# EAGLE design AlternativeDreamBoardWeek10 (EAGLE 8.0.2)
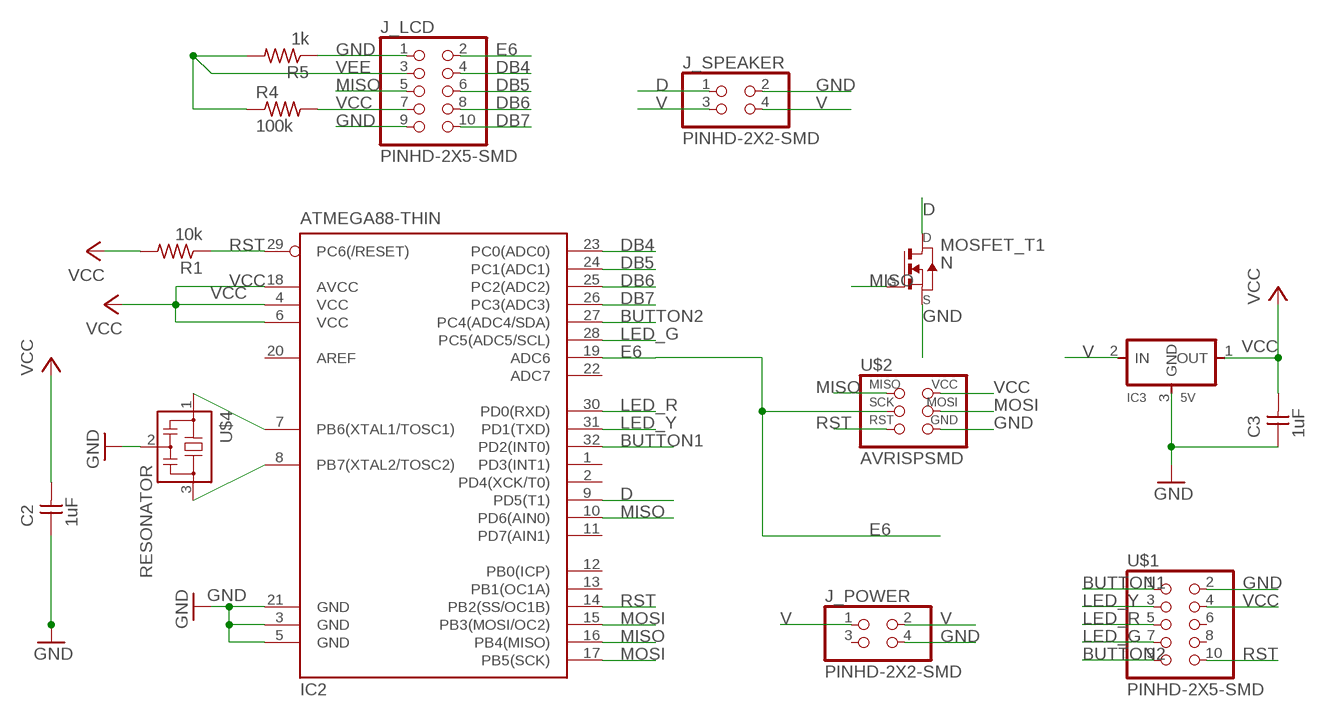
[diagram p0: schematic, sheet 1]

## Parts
C2  1uF  CAP-UNPOLARIZEDFAB  [C1206FAB]
C3  1uF  CAP-UNPOLARIZEDFAB  [C1206FAB]
IC2  ATMEGA88-THIN  [TQFP32-08THIN]
IC3  5V  REGULATORSOT23  [SOT23]
J_LCD  PINHD-2X5-SMD  [2X05SMD]
J_POWER  PINHD-2X2-SMD  [2X02SMD]
J_SPEAKER  PINHD-2X2-SMD  [2X02SMD]
MOSFET_T1  N  NMOSFETSOT23  [SOT-23]
R1  10k  RES-US1206FAB  [R1206FAB]
R4  100k  RES-US1206FAB  [R1206FAB]
R5  1k  RES-US1206FAB  [R1206FAB]
U$1  PINHD-2X5-SMD  [2X05SMD]
U$2  AVRISPSMD  [2X03SMD]
U$4  RESONATOR  [EFOBM]

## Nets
BUTTON1: IC2.32(PD2(INT0)) U$1.1
BUTTON2: IC2.27(PC4(ADC4/SDA)) U$1.9
D: IC2.9(PD5(T1)) J_SPEAKER.1 MOSFET_T1.1(D)
DB4: IC2.23(PC0(ADC0)) J_LCD.4
DB5: IC2.24(PC1(ADC1)) J_LCD.6
DB6: IC2.25(PC2(ADC2)) J_LCD.8
DB7: IC2.26(PC3(ADC3)) J_LCD.10
E6: IC2.19(ADC6) J_LCD.2 U$2.3(SCK)
GND: C2.1 C3.1 IC2.3(GND) IC2.5(GND) IC2.21(GND) IC3.3(GND) J_LCD.1 J_LCD.9 J_POWER.4 J_SPEAKER.2 MOSFET_T1.2(S) R5.1 U$1.2 U$2.6(GND) U$4.2
LED_G: IC2.28(PC5(ADC5/SCL)) U$1.7
LED_R: IC2.30(PD0(RXD)) U$1.5
LED_Y: IC2.31(PD1(TXD)) U$1.3
MISO: IC2.10(PD6(AIN0)) IC2.16(PB4(MISO)) J_LCD.5 MOSFET_T1.3(G) U$2.1(MISO)
MOSI: IC2.15(PB3(MOSI/OC2)) IC2.17(PB5(SCK)) U$2.4(MOSI)
N$1: IC2.8(PB7(XTAL2/TOSC2)) U$4.3
N$2: IC2.7(PB6(XTAL1/TOSC1)) U$4.1
RST: IC2.14(PB2(SS/OC1B)) IC2.29(PC6(/RESET)) R1.1 U$1.10 U$2.5(RST)
V: IC3.2(IN) J_POWER.1 J_POWER.2 J_SPEAKER.3 J_SPEAKER.4
VCC: C2.2 C3.2 IC2.4(VCC) IC2.6(VCC) IC2.18(AVCC) IC3.1(OUT) J_LCD.7 R1.2 R4.2 U$1.4 U$2.2(VCC)
VEE: J_LCD.3 R4.1 R5.2
Unconnected: IC2.1(PD3(INT1)) IC2.2(PD4(XCK/T0)) IC2.11(PD7(AIN1)) IC2.12(PB0(ICP)) IC2.13(PB1(OC1A)) IC2.20(AREF) IC2.22(ADC7) J_POWER.3 U$1.6 U$1.8

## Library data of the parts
C2 C3 = fab:CAP-UNPOLARIZED
IC2 = fab:ATMEGA88-THIN
IC3 = fab:REGULATOR
J_LCD U$1 = fab:PINHD-2X5-SMD
J_POWER J_SPEAKER = fab:PINHD-2X2-SMD
MOSFET_T1 = fab:NMOSFET: MOS FET
R1 R4 R5 = fab:RES-US: Resistor (US Symbol)
U$2 = fab:AVRISP
U$4 = fab:RESONATOR

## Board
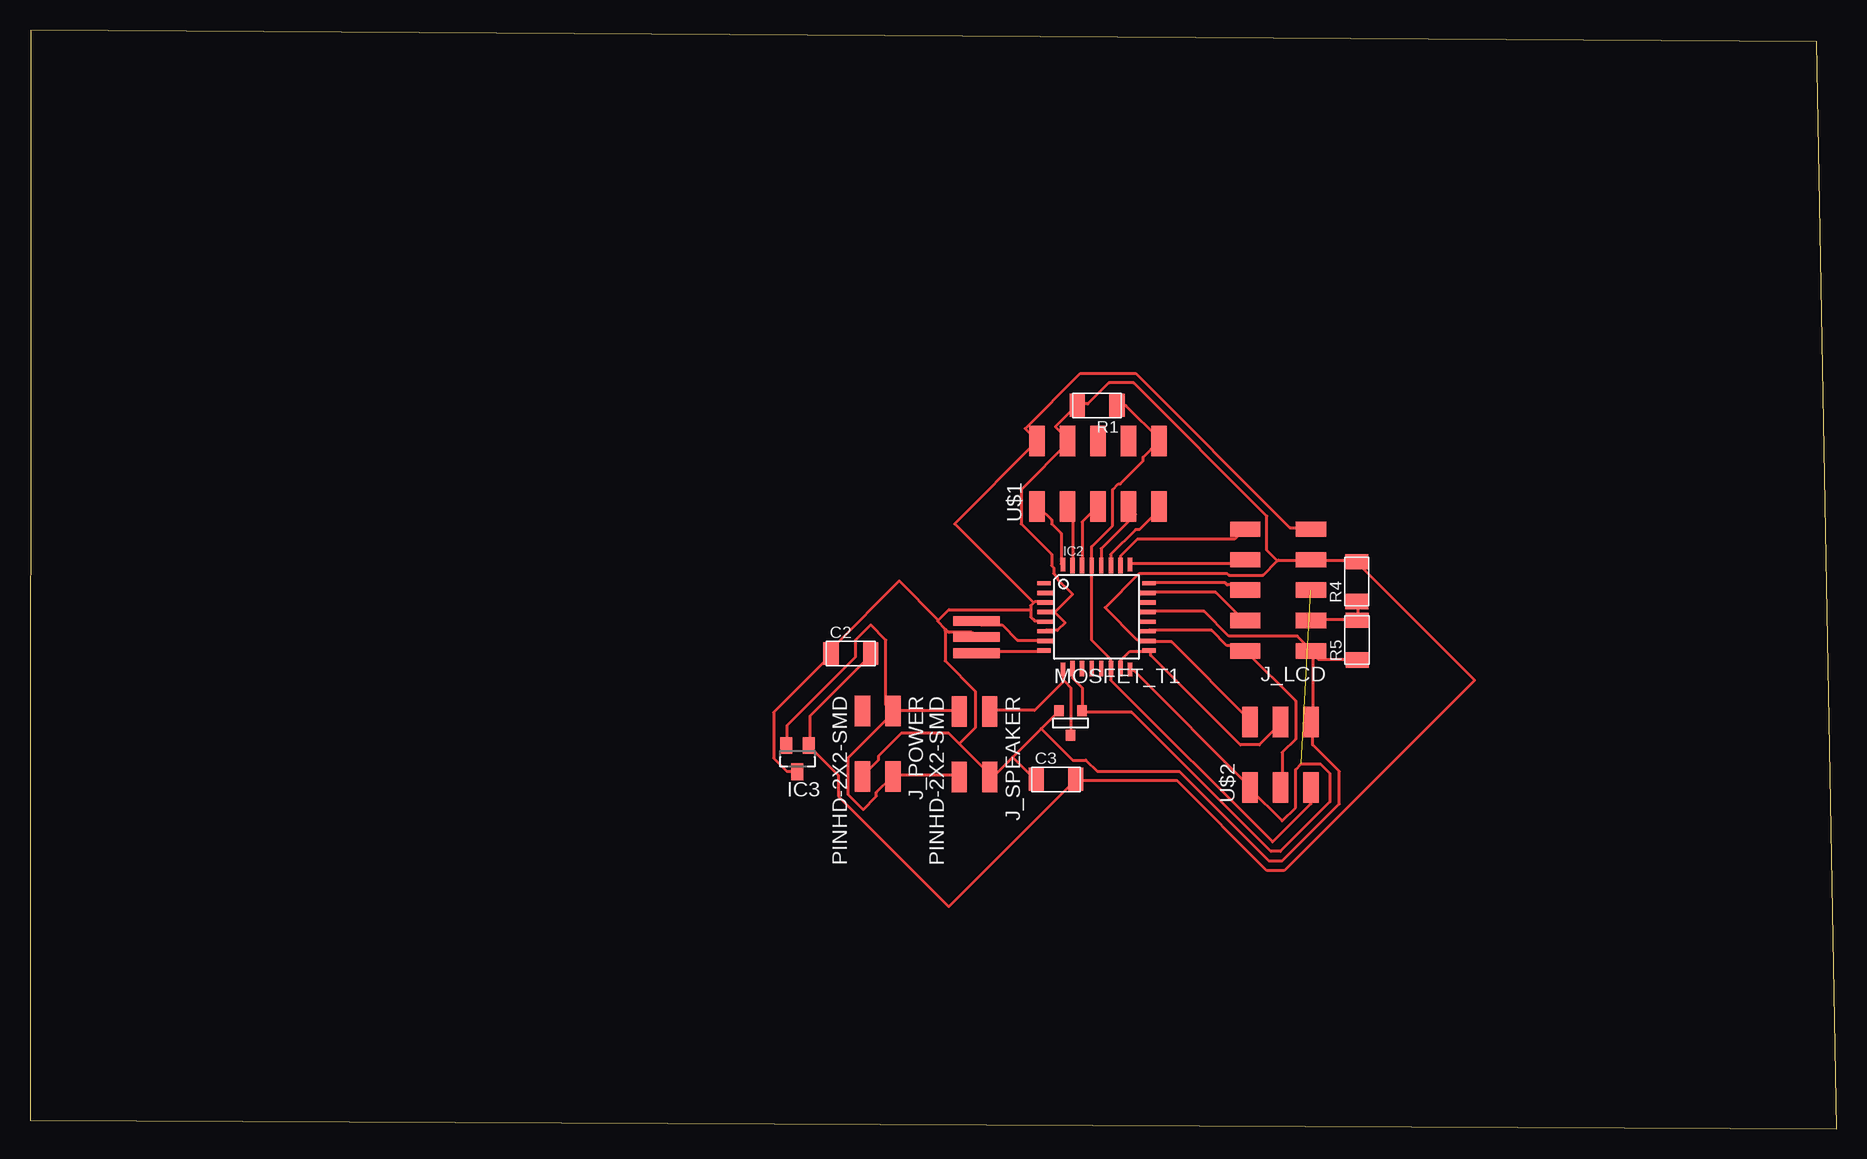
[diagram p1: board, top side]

Size 150.55 x 91.58 mm. Coordinates in mm from the lower left corner, seen from the top.
Outline: 0,0.71 150.55,0 148.89,90.62 0.08,91.58 0,0.71
Copper layers (1*16): Top 0.035mm / dielectric 1.5mm / Bottom 0.035mm
Design rules "default *": minimum track width 10mil, minimum drill 24mil, track to track 16mil, track to pad 16mil, pad to pad 16mil, via to via 16mil, smd to smd 8mil, copper to edge 40mil, drill to drill 8mil, minimum pad ring 10mil, minimum via ring 8mil, stop-mask expansion 4mil, vias tented up to drill 0mil, thermal gap 10mil

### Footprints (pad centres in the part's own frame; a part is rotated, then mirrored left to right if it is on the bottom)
C1206FAB = smd 1.27 x 1.905: 1 -1.651,0; 2 1.651,0
TQFP32-08THIN = smd 1.118 x 0.356: 1 -4.369,2.8; 8 -4.369,-2.8; 17 4.369,-2.8; 24 4.369,2.8 | smd 1.27 x 0.356: 2 -4.293,2; 3 -4.293,1.2; 4 -4.293,0.4; 5 -4.293,-0.4; 6 -4.293,-1.2; 7 -4.293,-2; 18 4.293,-2; 19 4.293,-1.2; 20 4.293,-0.4; 21 4.293,0.4; 22 4.293,1.2; 23 4.293,2 | smd 0.356 x 1.118: 9 -2.8,-4.369; 16 2.8,-4.369; 25 2.8,4.369; 32 -2.8,4.369 | smd 0.356 x 1.27: 10 -2,-4.293; 14 1.2,-4.293; 15 2,-4.293; 26 2,4.293; 27 1.2,4.293; 31 -2,4.293 | smd 0.35 x 1.27: 11 -1.2,-4.293; 12 -0.4,-4.293; 13 0.4,-4.293; 28 0.4,4.293; 29 -0.4,4.293; 30 -1.2,4.293
SOT23 = smd 1 x 1.4: 1 -0.95,-1.1; 2 0.95,-1.1; 3 0,1.1
2X05SMD = smd 2.54 x 1.27: 1 -2.54,2.54; 2 2.92,2.54; 3 -2.54,0; 4 2.92,0; 5 -2.54,-2.54; 6 2.92,-2.54; 7 -2.54,-5.08; 8 2.92,-5.08; 9 -2.54,-7.62; 10 2.92,-7.62
2X02SMD = smd 2.54 x 1.27: 1 -2.54,1.27; 2 2.92,1.27; 3 -2.54,-1.27; 4 2.92,-1.27
SOT-23 = smd 0.787 x 0.889: 1 0.025,-1.016; 2 -0.94,1.016; 3 0.991,1.016
R1206FAB = smd 1.27 x 1.905: 1 -1.651,0; 2 1.651,0
2X03SMD = smd 2.54 x 1.27: 1 -2.54,2.54; 2 2.92,2.54; 3 -2.54,0; 4 2.92,0; 5 -2.54,-2.54; 6 2.92,-2.54
EFOBM = smd 0.8 x 3.9: 1 -1.35,0; 2 0,0; 3 1.35,0

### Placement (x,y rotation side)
C2  68.4,39.62 0 top
C3  85.5,29.13 0 top
IC2  88.87,42.67 0 top
IC3  63.96,30.86 180 top
J_LCD  104.19,42.37 180 top
J_POWER  70.64,32.28 270 top
J_SPEAKER  78.71,32.26 270 top
MOSFET_T1  86.69,33.83 0 top
R1  88.93,60.3 180 top
R4  110.57,45.62 90 top
R5  110.59,40.74 90 top
U$1  86.46,54.41 90 top
U$2  104.22,31.01 90 top
U$4  78.87,41 270 top

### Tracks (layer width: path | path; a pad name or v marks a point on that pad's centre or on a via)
BUTTON1
  Top 0.254: IC2.32 85.93,47.1 85.93,49.64 85.14,50.43 85.14,50.75 84.03,51.86 U$1.1
BUTTON2
  Top 0.254: IC2.27 90.06,47.1 90.06,47.89 92.13,49.96 92.44,49.96 94.19,51.7 94.03,51.86 U$1.9
D
  Top 0.254: 86.17,37.34 86.09,37.41 86.09,38.21 IC2.9 | 86.17,37.34 86.73,36.78 86.73,32.97 MOSFET_T1.1 | 86.17,37.34 83.71,34.87 80.06,34.87 J_SPEAKER.1
DB4
  Top 0.254: IC2.23 93.24,44.72 98.79,44.72 101.17,42.34 J_LCD.4
DB5
  Top 0.254: IC2.24 93.4,45.51 99.59,45.51 99.75,45.35 100.86,45.35 101.17,45.03 J_LCD.6
DB6
  Top 0.254: IC2.25 91.81,47.1 100.86,47.1 101.17,47.42 J_LCD.8
DB7
  Top 0.254: IC2.26 90.86,47.1 90.86,47.73 92.28,49.16 100.38,49.16 101.17,49.96 J_LCD.10
E6
  Top 0.254: IC2.19 93.24,41.54 98.48,41.54 99.75,40.27 100.86,40.27 101.17,39.95 J_LCD.2 101.33,39.8 105.46,35.67 105.46,32.49 104.35,31.38 104.35,28.52 U$2.3
GND
  Top 0.254: IC2.21 93.24,43.13 97.84,43.13 99.9,41.07 105.62,41.07 106.73,39.95 J_LCD.1 | R5.1 110.54,39.16 107.37,39.16 106.73,39.8 J_LCD.1 | J_LCD.1 106.89,39.48 106.89,34.08 U$2.6 106.89,33.92 106.89,32.02 109.11,29.79 109.11,27.1 104.35,22.33 103.24,22.33 95.78,29.79 88.95,29.79 88,30.75 86.89,30.75 84.27,33.37 | 81.89,30.99 80.22,29.32 80.06,29.48 | 81.89,30.99 84.27,33.37 | 84.27,33.37 MOSFET_T1.2 | 81.89,30.99 83.71,29.16 C3.1 | 80.06,29.48 77.44,32.1 | 77.44,32.1 76.57,32.97 72.6,32.97 70.69,31.06 70.69,30.75 69.42,29.48 J_POWER.4 | 80.06,29.48 J_SPEAKER.2 | IC3.3 63.87,29.79 63.07,29.79 61.96,30.91 61.96,34.72 66.73,39.48 C2.1 66.88,39.64 66.88,40.11 72.44,45.67 75.69,42.42 | 83.39,43.29 83.39,43.61 83.63,43.84 | 83.39,43.29 83.39,42.65 83.71,42.34 84.51,42.34 IC2.5 | 83.63,43.84 83.71,43.92 84.51,43.92 IC2.3 | 83.39,43.29 76.57,43.29 75.69,42.42 | 75.69,42.42 75.62,42.34 76.33,41.62 | 76.33,41.62 76.57,41.38 78.47,41.38 78.79,41.07 U$4.2 | 83.63,43.84 77.04,50.43 83.87,57.26 U$1.2 83.87,57.42 82.92,58.37 87.52,62.97 92.13,62.97 104.98,50.11 106.73,50.11 J_LCD.9 | 77.44,32.1 78.79,33.45 78.79,36.46 76.25,39 76.25,41.54 76.33,41.62
LED_G
  Top 0.254: IC2.28 89.27,47.1 89.27,48.37 92.13,51.23 91.49,51.86 U$1.7
LED_R
  Top 0.254: IC2.30 87.68,47.1 87.68,50.59 88.95,51.86 U$1.5
LED_Y
  Top 0.254: IC2.31 86.89,47.1 86.89,51.54 86.57,51.86 U$1.3
MISO  (1 unrouted)
  Top 0.254: IC2.10 86.89,38.37 86.89,37.57 87.68,36.78 MOSFET_T1.3 87.68,34.72 91.81,34.72 103.4,23.13 104.19,23.13 108.32,27.25 108.32,29.64 107.52,30.43 105.94,30.43 105.46,29.95 105.46,26.78 104.35,25.67 101.65,28.37 U$2.1 101.65,28.52 91.97,38.21 91.81,38.21 IC2.16
MOSI
  Top 0.254: IC2.15 90.86,38.53 90.86,39 91.65,39.8 93.24,39.8 IC2.17 93.4,39.8 93.4,39.48 100.86,32.02 102.44,32.02 104.35,33.92 U$2.4
N$1
  Top 0.254: IC2.8 84.51,39.8 78.95,39.8 U$4.3
N$2
  Top 0.254: IC2.7 84.51,40.75 82.28,40.75 81.01,42.02 79.27,42.02 78.95,42.34 U$4.1
RST
  Top 0.254: R1.1 90.7,60.27 91.33,60.27 94.19,57.42 U$1.10 94.03,57.26 92.76,55.99 92.76,55.67 90.86,53.77 90.7,53.77 90.22,53.29 90.22,50.27 88.47,48.53 88.47,47.1 IC2.29 88.47,46.94 88.47,40.75 90.06,39.16 90.06,38.53 IC2.14 90.06,38.37 90.06,37.41 103.56,23.92 106.73,27.1 106.73,28.37 U$2.5
V
  Top 0.254: J_SPEAKER.4 77.36,29.48 71.96,29.48 J_POWER.2 71.81,29.32 70.54,28.05 70.54,27.73 69.42,26.62 68.15,27.89 68.15,30.91 71.96,34.72 J_POWER.1 | IC3.2 63.07,32.02 63.07,33.6 68.79,39.32 68.79,40.75 70.06,42.02 71.33,40.75 71.33,35.35 71.81,34.87 J_POWER.1 | J_SPEAKER.3 77.36,34.87 71.96,34.87 J_POWER.1
VCC
  Top 0.254: C2.2 70.06,39.48 64.98,34.4 64.98,32.02 IC3.1 64.98,31.86 67.36,29.48 67.36,27.73 76.57,18.52 87.05,29 C3.2 87.2,29 95.62,29 103.08,21.54 104.51,21.54 120.38,37.41 110.54,47.26 R4.2 110.54,47.42 106.73,47.42 | 85.38,43.05 85.3,43.13 84.66,43.13 IC2.4 | 85.38,43.05 86.25,42.18 85.62,41.54 84.66,41.54 IC2.6 | 85.38,43.05 86.89,44.56 85.62,45.83 85.62,45.99 85.3,46.3 85.3,46.78 85.14,46.94 85.14,47.89 82.6,50.43 82.6,53.29 86.57,57.26 U$1.4 86.57,57.42 85.46,58.53 87.2,60.27 R1.2 87.36,60.43 88.16,60.43 89.9,62.18 91.97,62.18 103.08,51.07 103.08,48.21 103.95,47.34 | U$2.2 101.65,34.08 95.14,40.59 93.24,40.59 IC2.18 93.08,40.75 92.28,40.75 89.59,43.45 92.44,46.3 99.75,46.3 99.9,46.15 102.76,46.15 103.95,47.34 | 106.73,47.42 104.03,47.42 103.95,47.34 | 106.73,47.42 J_LCD.7
VEE
  Top 0.254: R4.1 110.7,43.92 110.7,42.49 R5.2 110.54,42.49 106.73,42.49 J_LCD.3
